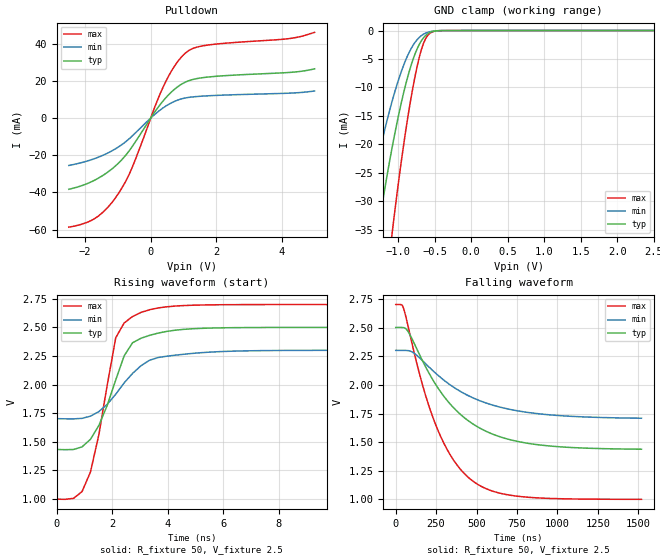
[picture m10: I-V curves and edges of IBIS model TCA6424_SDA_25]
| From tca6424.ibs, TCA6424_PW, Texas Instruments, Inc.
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[Model]   TCA6424_SDA_25
Model_type  I/O_open_drain
Vinl=0.69
Vinh=1.89
Enable   Active-Low
Vref =   0
Rref =   500
Cref =   50p
Vmeas =   1.25
| variable   typ   min   max
C_comp   3.07pF   2.08pF   3.53pF
| C_pulldown   1.93pF   0.76pF   2.66pF
| C_tri-state   3.07pF   2.08pF   3.53pF
[Temperature Range]   40   100   -40
| Ambient temperature   25   85   -40
[Voltage range]   2.5   2.3   2.7
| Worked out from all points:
|   slope of the pulldown table from 0 to 0.375 V, typ, clamps not added: 41 ohm
|   GND clamp passes 1 mA (typ) near -0.63 V on its own axis
|   rising waveform, R_fixture 50, V_fixture 2.5: 20-80 % time 996ps typ, 1.34ns min, 777ps max; typ from 1.44 V to 2.5 V
|   falling waveform, R_fixture 50, V_fixture 2.5: 20-80 % time 347ns typ, 404ns min, 258ns max; typ from 2.5 V to 1.44 V
[GND Clamp]
| TCA6424_SDA_25
|   Voltage   I(typ)   I(min)   I(max)
-2.5V     -164.8mA   -119.5mA   -236.9mA
-1.49V    -54.18mA   -36.17mA   -85.83mA
-1.46V    -51.4mA    -34.15mA   -81.8mA
-1.27V    -34.83mA   -22.3mA    -57.41mA
-1.08V    -20.52mA   -12.39mA   -35.53mA
-955mV    -12.69mA   -7.213mA   -22.99mA
-835mV    -6.702mA   -3.527mA   -12.83mA
-725mV    -2.857mA   -1.42mA    -5.559mA
-645mV    -1.188mA   -600.5uA   -2.074mA
-570mV    -395.1uA   -226.1uA   -548.7uA
-435mV    -28.55uA   -22.65uA   -25.45uA
2.5V      291.4pA    899.7pA    103.8pA
[Pulldown]
| TCA6424_SDA_25
|   Voltage   I(typ)   I(min)   I(max)
-2.5V     -38.28mA   -25.48mA   -58.63mA
-1.665V   -32.94mA   -21.48mA   -53.47mA
-1.325V   -29.22mA   -18.91mA   -48.24mA
-1.005V   -24.56mA   -15.75mA   -41.05mA
-585mV    -15.83mA   -9.951mA   -27.3mA
150mV     3.947mA    2.363mA    7.134mA
425mV     10.19mA    6.023mA    18.39mA
760mV     15.97mA    9.213mA    28.81mA
1.09V     19.56mA    10.9mA     35.38mA
1.67V     21.89mA    11.89mA    39.05mA
4.19V     24.47mA    13.35mA    42.64mA
5V        26.46mA    14.57mA    46.07mA
[Ramp]
| TCA6424_SDA_25
| variable   typ   min   max
dV/dt_r   0.64/9.78E-10   0.36/1.33E-09   1.02/7.53E-10
dV/dt_f   0.64/3.47E-07   0.36/4.04E-07   1.02/2.58E-07
R_load = 50
[Rising Waveform]
| TCA6424_SDA_25
R_fixture =   50
C_fixture =   0
L_fixture =   0
V_fixture =   2.5
V_fixture_min = 2.3
V_fixture_max = 2.7
|   Time   V(typ)   V(min)   V(max)
0s        1.435V     1.704V     1.001V
917ps     1.455V     1.705V     1.064V
1.221ns   1.521V     1.724V     1.235V
1.525ns   1.643V     1.764V     1.562V
2.133ns   2.041V     1.916V     2.409V
2.437ns   2.252V     2.015V     2.539V
2.741ns   2.366V     2.098V     2.595V
3.653ns   2.45V      2.236V     2.67V
6.389ns   2.497V     2.292V     2.699V
1.52us    2.5V       2.3V       2.7V
[Falling Waveform]
| TCA6424_SDA_25
R_fixture =   50
C_fixture =   0
L_fixture =   0
V_fixture =   2.5
V_fixture_min = 2.3
V_fixture_max = 2.7
|   Time   V(typ)   V(min)   V(max)
0s        2.5V       2.3V       2.7V
48.65ns   2.499V     2.301V     2.667V
82.69ns   2.451V     2.297V     2.474V
168.1ns   2.204V     2.208V     1.988V
267.5ns   1.96V      2.076V     1.583V
361.8ns   1.795V     1.976V     1.335V
468.8ns   1.667V     1.892V     1.168V
613.5ns   1.563V     1.818V     1.067V
826.9ns   1.488V     1.758V     1.018V
1.52us    1.438V     1.709V     1.001V
